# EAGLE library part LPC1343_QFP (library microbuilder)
LPC1343 72 MHz 32-bit ARM Cortex-M3 microcontroller. 32 kB Flash, 8 kB SRAM, USB Device Mouser: 771-LPC1343FBD48151 Digikey: 568-4945-ND
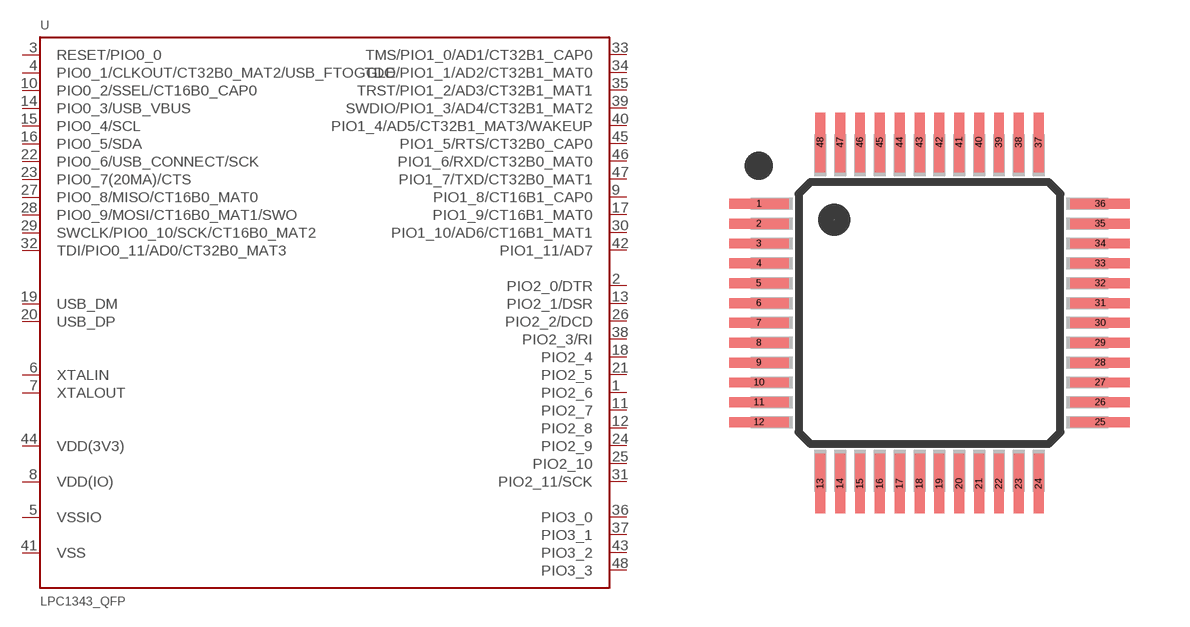
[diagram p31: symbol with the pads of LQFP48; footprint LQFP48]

Designator prefix U

## LPC1343_QFP (DIGIKEY#: 568-4945-ND; MANF: NXP; MANF#: LPC1343FBD48,151)  [LQFP48]
1  PIO2_6
2  PIO2_0/DTR
3  RESET/PIO0_0
4  PIO0_1/CLKOUT/CT32B0_MAT2/USB_FTOGGLE
5  VSSIO  pwr
6  XTALIN  in
7  XTALOUT  out
8  VDD(IO)  pwr
9  PIO1_8/CT16B1_CAP0
10  PIO0_2/SSEL/CT16B0_CAP0
11  PIO2_7
12  PIO2_8
13  PIO2_1/DSR
14  PIO0_3/USB_VBUS
15  PIO0_4/SCL
16  PIO0_5/SDA
17  PIO1_9/CT16B1_MAT0
18  PIO2_4
19  USB_DM
20  USB_DP
21  PIO2_5
22  PIO0_6/USB_CONNECT/SCK
23  PIO0_7(20MA)/CTS
24  PIO2_9
25  PIO2_10
26  PIO2_2/DCD
27  PIO0_8/MISO/CT16B0_MAT0
28  PIO0_9/MOSI/CT16B0_MAT1/SWO
29  SWCLK/PIO0_10/SCK/CT16B0_MAT2
30  PIO1_10/AD6/CT16B1_MAT1
31  PIO2_11/SCK
32  TDI/PIO0_11/AD0/CT32B0_MAT3
33  TMS/PIO1_0/AD1/CT32B1_CAP0
34  TDO/PIO1_1/AD2/CT32B1_MAT0
35  TRST/PIO1_2/AD3/CT32B1_MAT1
36  PIO3_0
37  PIO3_1
38  PIO2_3/RI
39  SWDIO/PIO1_3/AD4/CT32B1_MAT2
40  PIO1_4/AD5/CT32B1_MAT3/WAKEUP
41  VSS  pwr
42  PIO1_11/AD7
43  PIO3_2
44  VDD(3V3)  pwr
45  PIO1_5/RTS/CT32B0_CAP0
46  PIO1_6/RXD/CT32B0_MAT0
47  PIO1_7/TXD/CT32B0_MAT1
48  PIO3_3

## Footprint LQFP48 (pad centres in mm)
smd 1.5 x 0.25: 1 -4.3,2.75; 2 -4.3,2.25; 3 -4.3,1.75; 4 -4.3,1.25; 5 -4.3,0.75; 6 -4.3,0.25; 7 -4.3,-0.25; 8 -4.3,-0.75; 9 -4.3,-1.25; 10 -4.3,-1.75; 11 -4.3,-2.25; 12 -4.3,-2.75; 25 4.3,-2.75; 26 4.3,-2.25; 27 4.3,-1.75; 28 4.3,-1.25; 29 4.3,-0.75; 30 4.3,-0.25; 31 4.3,0.25; 32 4.3,0.75; 33 4.3,1.25; 34 4.3,1.75; 35 4.3,2.25; 36 4.3,2.75
smd 0.25 x 1.5: 13 -2.75,-4.3; 14 -2.25,-4.3; 15 -1.75,-4.3; 16 -1.25,-4.3; 17 -0.75,-4.3; 18 -0.25,-4.3; 19 0.25,-4.3; 20 0.75,-4.3; 21 1.25,-4.3; 22 1.75,-4.3; 23 2.25,-4.3; 24 2.75,-4.3; 37 2.75,4.3; 38 2.25,4.3; 39 1.75,4.3; 40 1.25,4.3; 41 0.75,4.3; 42 0.25,4.3; 43 -0.25,4.3; 44 -0.75,4.3; 45 -1.25,4.3; 46 -1.75,4.3; 47 -2.25,4.3; 48 -2.75,4.3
